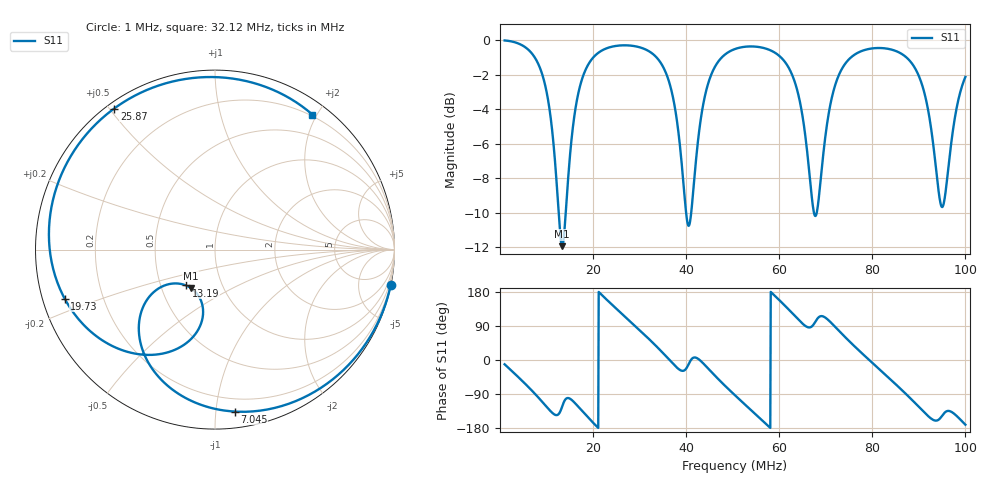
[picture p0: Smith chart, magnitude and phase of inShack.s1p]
# MHz S RI R 50.0
! SimSmith 18.4g
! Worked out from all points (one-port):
!   1000 points, 1 MHz to 100 MHz, reference 50 ohm
!   lowest |S11| = -11.9 dB at 13.39 MHz (marker M1), VSWR 1.68, Z = 35.1 - j16.1 ohm
!   |S11| at or under -10 dB: 12.61 MHz to 14.14 MHz (1.529 MHz wide, 11.4 % of centre); 39.99 MHz to 41.09 MHz (1.097 MHz wide, 2.71 % of centre); 67.46 MHz to 68.06 MHz (595.2 kHz wide, 0.878 % of centre)
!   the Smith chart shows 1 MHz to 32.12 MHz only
!   S11 on the Smith chart (normalised r, x): 1 MHz: 0, -10; 7.045 MHz: 0.11, -1.12; 13.19 MHz: 0.67, -0.29; 19.73 MHz: 0.06, -0.16; 25.87 MHz: 0.02, +0.51; 32.12 MHz: 0.18, +1.94
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1  0.9794 -0.196
7.045045  0.1099 -0.9025
10.41441  -0.4162 -0.5146
13.18919  -0.1612 -0.1999
13.38739  -0.1342 -0.2143
16.65766  -0.3513 -0.5864
19.72973  -0.8379 -0.2727
25.77478  -0.5767 0.7748
25.87387  -0.5616 0.7861
32.11712  0.5423 0.7526
35.28829  0.7972 0.2134
38.16216  0.5262 -0.2087
40.44144  0.2826 -0.0674
42.22523  0.4622 0.0453
45.49549  0.6764 -0.4293
50.54955  -0.061 -0.9419
57.18919  -0.9277 -0.1823
62.93694  -0.4127 0.6667
65.61261  0.000628 0.5276
67.79279  -0.0617 0.3031
70.66667  -0.1508 0.5984
75.32432  0.6147 0.6432
80.97297  0.9011 -0.2993
87.71171  -0.0831 -0.878
91.27928  -0.5297 -0.4514
94.94595  -0.2788 -0.1738
97.52252  -0.4455 -0.358
100  -0.7728 -0.1263
